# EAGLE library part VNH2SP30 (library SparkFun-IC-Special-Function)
30A motor driver IC(IC-10030,moster moto)
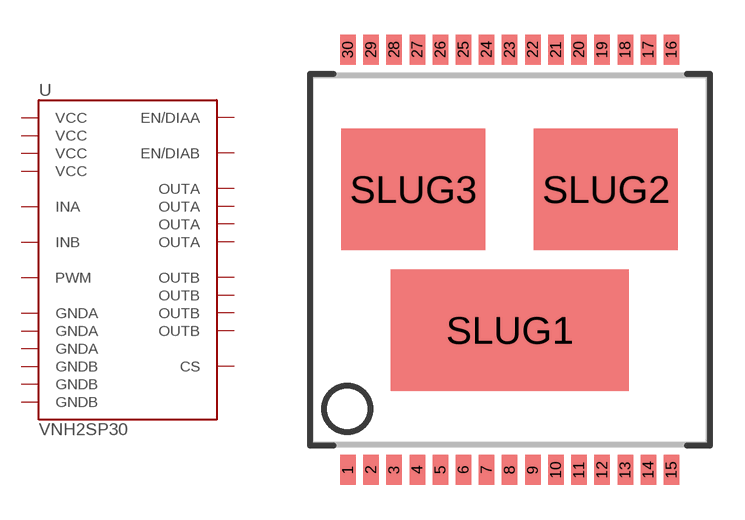
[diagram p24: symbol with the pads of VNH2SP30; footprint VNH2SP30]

Designator prefix -

## VNH2SP30  [VNH2SP30]
1  OUTA
3  VCC
5  INA
6  EN/DIAA
8  PWM
9  CS
10  EN/DIAB
11  INB
13  VCC
15  OUTB
16  OUTB
18  GNDB
19  GNDB
20  GNDB
21  OUTB
23  VCC
25  OUTA
26  GNDA
27  GNDA
28  GNDA
30  OUTA
SLUG1  VCC
SLUG2  OUTB
SLUG3  OUTA

## Footprint VNH2SP30 (pad centres in mm)
smd 0.67 x 1.3: 1 -7,-9.1; 2 -6,-9.1; 3 -5,-9.1; 4 -4,-9.1; 5 -3,-9.1; 6 -2,-9.1; 7 -1,-9.1; 8 0,-9.1; 9 1,-9.1; 10 2,-9.1; 11 3,-9.1; 12 4,-9.1; 13 5,-9.1; 14 6,-9.1; 15 7,-9.1; 16 7,9.1; 17 6,9.1; 18 5,9.1; 19 4,9.1; 20 3,9.1; 21 2,9.1; 22 1,9.1; 23 0,9.1; 24 -1,9.1; 25 -2,9.1; 26 -3,9.1; 27 -4,9.1; 28 -5,9.1; 29 -6,9.1; 30 -7,9.1
smd 10.3 x 5.25: SLUG1 0,-3.05
smd 6.23 x 5.25: SLUG2 4.165,3.05; SLUG3 -4.165,3.05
